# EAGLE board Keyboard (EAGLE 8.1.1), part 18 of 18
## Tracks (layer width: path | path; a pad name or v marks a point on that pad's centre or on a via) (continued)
S$18700 (continued)
  Bottom 0.381: 271.04,2.46 269.52,3.98
S$18701
  Bottom 0.381: 294.75,2.46 288.9,2.46
S$18702
  Bottom 0.381: 288.9,2.46 287.38,3.98
S$18703
  Bottom 0.381: 315.08,12.62 315.08,13.89
S$18704
  Bottom 0.381: 315.08,13.89 313.34,15.63
S$18705
  Bottom 0.381: 313.34,15.63 313.34,15.89
S$18706
  Bottom 0.381: 315.08,88.82 315.08,87.55
S$18707
  Bottom 0.381: 315.08,87.55 312.29,84.76
S$18708
  Bottom 0.381: 312.29,84.76 312.29,76.47
S$18709
  Bottom 0.381: 312.29,76.47 313.34,75.42
S$18710
  Bottom 0.381: 296.03,69.77 296.03,71.04
S$18711
  Bottom 0.381: 296.03,71.04 294.29,72.77
S$18712
  Bottom 0.381: 294.29,72.77 294.29,73.04
S$18713
  Bottom 0.381: 296.03,12.62 296.03,13.89
S$18714
  Bottom 0.381: 296.03,13.89 294.29,15.63
S$18715
  Bottom 0.381: 294.29,15.63 294.29,15.89
S$18716
  Bottom 0.381: 315.08,69.77 315.08,71.04
S$18717
  Bottom 0.381: 315.08,71.04 313.34,72.77
S$18718
  Bottom 0.381: 313.34,72.77 313.34,73.04
S$18719
  Bottom 0.381: 193.31,23.03 198.78,23.03
S$18720
  Bottom 0.381: 198.78,23.03 200.28,21.53
S$18721
  Bottom 0.381: 294.76,21.51 290.09,21.51
S$18722
  Bottom 0.381: 290.09,21.51 288.56,23.03
S$18723
  Bottom 0.381: 268.22,69.78 269.49,69.78
S$18724
  Bottom 0.381: 269.49,69.78 269.49,69.22
S$18725
  Bottom 0.381: 269.49,69.22 270.2,68.51
S$18726
  Bottom 0.381: 270.2,68.51 277.86,68.51
S$18727
  Bottom 0.381: 179.02,61.13 184.49,61.13
S$18728
  Bottom 0.381: 184.49,61.13 185.99,59.63
S$18729
  Bottom 0.381: 254.04,58.75 244.01,58.75
S$18730
  Bottom 0.381: 244.01,58.75 243.14,59.62
S$18731
  Bottom 0.381: 174.26,30.65 168.98,30.65
S$18732
  Bottom 0.381: 168.98,30.65 166.68,32.95
S$18733
  Bottom 0.381: 166.68,32.95 165.41,32.95
S$18734
  Bottom 0.381: 165.41,32.95 164.71,32.24
S$18735
  Bottom 0.381: 164.71,32.24 164.71,30.54
S$18736
  Bottom 0.381: 164.71,30.54 164.45,30.28
S$18737
  Bottom 0.381: 164.45,30.28 155.57,30.28
S$18738
  Bottom 0.381: 155.57,30.28 155.21,30.65
S$18739
  Bottom 0.381: 98.05,30.65 97.7,30.29
S$18740
  Bottom 0.381: 97.7,30.29 79.35,30.29
S$18741
  Bottom 0.381: 79.35,30.29 79,30.65
S$18742
  Bottom 0.381: 136.15,30.65 135.77,30.26
S$18743
  Bottom 0.381: 135.77,30.26 117.49,30.26
S$18744
  Bottom 0.381: 117.49,30.26 117.1,30.65
S$18745
  Bottom 0.381: 155.21,23.03 160.68,23.03
S$18746
  Bottom 0.381: 160.68,23.03 162.18,21.52
S$18747
  Bottom 0.381: 144.4,31.69 144.4,32.96
S$18748
  Bottom 0.381: 144.4,32.96 143.85,32.96
S$18749
  Bottom 0.381: 143.85,32.96 141.87,34.94
S$18750
  Bottom 0.381: 294.75,59.61 290.09,59.61
S$18751
  Bottom 0.381: 290.09,59.61 288.57,61.13
S$18752
  Bottom 0.381: 294.75,78.66 293,78.66
S$18753
  Bottom 0.381: 293,78.66 287.39,73.04
S$18754
  Bottom 0.381: 283.78,80.82 286.22,83.26
S$18755
  Bottom 0.381: 286.22,83.26 286.22,83.42
S$18756
  Bottom 0.381: 45.66,61.13 51.14,61.13
S$18757
  Bottom 0.381: 51.14,61.13 52.64,59.63
S$18758
  Bottom 0.381: 69.47,42.08 74.95,42.08
S$18759
  Bottom 0.381: 74.95,42.08 76.45,40.57
S$18760
  Bottom 0.381: 313.8,2.46 298.98,2.46
S$18761
  Bottom 0.381: 298.98,2.46 298.55,2.89
S$18762
  Bottom 0.381: 298.55,2.89 297.76,2.89
S$18763
  Bottom 0.381: 297.76,2.89 296.91,3.74
S$18764
  Bottom 0.381: 296.91,3.74 296.91,3.98
S$18765
  Bottom 0.381: 296.91,3.98 289.76,3.98
S$18766
  Bottom 0.381: 297.57,77.69 297,77.12
S$18767
  Bottom 0.381: 297,77.12 293.85,77.12
S$18768
  Bottom 0.381: 293.85,77.12 289.77,73.04
S$18769
  Bottom 0.381: 307.63,61.13 309.14,59.61
S$18770
  Bottom 0.381: 309.14,59.61 309.35,59.61
S$18771
  Bottom 0.381: 50.42,42.08 55.9,42.08
S$18772
  Bottom 0.381: 55.9,42.08 57.41,40.57
S$18773
  Bottom 0.381: 25.42,2.78 23.62,0.99
S$18774
  Bottom 0.381: 23.62,0.99 8.88,0.99
S$18775
  Bottom 0.381: 8.88,0.99 7.4,2.47
S$18776
  Bottom 0.381: 246.8,12.63 248.07,12.63
S$18777
  Bottom 0.381: 248.07,12.63 248.07,12
S$18778
  Bottom 0.381: 248.07,12 248.7,11.36
S$18779
  Bottom 0.381: 248.7,11.36 255.24,11.36
S$18780
  Bottom 0.381: 255.24,11.36 256.43,12.55
S$18781
  Bottom 0.381: 280.76,26.2 281.42,25.55
S$18782
  Bottom 0.381: 281.42,25.55 281.42,22.81
S$18783
  Bottom 0.381: 272.86,24.62 272.09,25.39
S$18784
  Bottom 0.381: 272.09,25.39 272.09,29.48
S$18785
  Bottom 0.381: 272.09,29.48 272.2,29.6
S$18786
  Bottom 0.381: 272.2,29.6 277.37,29.6
S$18787
  Bottom 0.381: 277.37,29.6 280.76,26.2
S$18788
  Bottom 0.381: 280.76,26.2 284.99,30.43
S$18789
  Bottom 0.381: 272.86,23.03 272.86,24.62
S$18790
  Bottom 0.381: 220.6,31.69 220.6,32.96
S$18791
  Bottom 0.381: 220.6,32.96 220.06,32.96
S$18792
  Bottom 0.381: 220.06,32.96 218.08,34.94
S$18793
  Bottom 0.381: 201.55,31.69 201.55,32.96
S$18794
  Bottom 0.381: 201.55,32.96 201.01,32.96
S$18795
  Bottom 0.381: 201.01,32.96 199.03,34.94
S$18796
  Bottom 0.381: 225.36,69.78 225.36,71.05
S$18797
  Bottom 0.381: 225.36,71.05 224.83,71.05
S$18798
  Bottom 0.381: 224.83,71.05 222.84,73.04
S$18799
  Bottom 0.381: 39.62,50.74 39.62,52.01
S$18800
  Bottom 0.381: 39.62,52.01 39.07,52.01
S$18801
  Bottom 0.381: 39.07,52.01 37.09,53.99
S$18802
  Bottom 0.381: 82.49,88.83 82.49,87.56
S$18803
  Bottom 0.381: 82.49,87.56 79.64,84.71
S$18804
  Bottom 0.381: 79.64,84.71 79.64,75.73
S$18805
  Bottom 0.381: 79.64,75.73 79.95,75.42
S$18806
  Bottom 0.381: 87.25,31.68 87.25,32.95
S$18807
  Bottom 0.381: 84.72,34.94 86.7,32.95
S$18808
  Bottom 0.381: 86.7,32.95 87.25,32.95
S$18809
  Bottom 0.381: 77.72,50.73 77.72,52
S$18810
  Bottom 0.381: 77.72,52 77.18,52
S$18811
  Bottom 0.381: 77.18,52 75.19,53.99
S$18812
  Bottom 0.381: 164.74,42.08 170.2,42.08
S$18813
  Bottom 0.381: 170.2,42.08 171.7,40.57
S$18814
  Bottom 0.381: 183.79,42.08 189.25,42.08
S$18815
  Bottom 0.381: 189.25,42.08 190.75,40.58
S$18816
  Bottom 0.381: 211.07,50.74 211.07,52.01
S$18817
  Bottom 0.381: 211.07,52.01 210.54,52.01
S$18818
  Bottom 0.381: 210.54,52.01 208.55,53.98
S$18819
  Bottom 0.381: 221.89,42.08 223.39,40.58
S$18820
  Bottom 0.381: 223.39,40.58 228.85,40.58
S$18821
  Bottom 0.381: 261.08,50.73 261.08,52
S$18822
  Bottom 0.381: 261.08,52 260.56,52
S$18823
  Bottom 0.381: 260.56,52 258.57,53.99
S$18824
  Bottom 0.381: 49.15,31.69 49.15,32.96
S$18825
  Bottom 0.381: 49.15,32.96 48.59,32.96
S$18826
  Bottom 0.381: 48.59,32.96 46.61,34.94
S$18827
  Bottom 0.381: 42.09,23.03 46.38,23.03
S$18828
  Bottom 0.381: 46.38,23.03 47.88,21.53
S$18829
  Bottom 0.381: 68.2,31.68 68.2,32.95
S$18830
  Bottom 0.381: 68.2,32.95 67.65,32.95
S$18831
  Bottom 0.381: 67.65,32.95 65.66,34.94
S$18832
  Bottom 0.381: 59.94,23.03 65.42,23.03
S$18833
  Bottom 0.381: 65.42,23.03 66.93,21.52
S$18834
  Bottom 0.381: 153.92,50.73 153.92,52
S$18835
  Bottom 0.381: 153.92,52 153.39,52
S$18836
  Bottom 0.381: 153.39,52 151.4,53.99
S$18837
  Bottom 0.381: 126.62,42.08 132.1,42.08
S$18838
  Bottom 0.381: 132.1,42.08 133.6,40.57
S$18839
  Bottom 0.381: 79,23.03 84.47,23.03
S$18840
  Bottom 0.381: 84.47,23.03 85.98,21.52
S$18841
  Bottom 0.381: 44.47,3.98 43.34,5.11
S$18842
  Bottom 0.381: 43.34,5.11 41.17,5.11
S$18843
  Bottom 0.381: 41.17,5.11 38.54,2.48
S$18844
  Bottom 0.381: 38.54,2.48 31.21,2.48
S$18845
  Bottom 0.381: 56.29,12.64 56.29,13.91
S$18846
  Bottom 0.381: 56.29,13.91 55.74,13.91
S$18847
  Bottom 0.381: 55.74,13.91 53.76,15.89
S$18848
  Bottom 0.381: 49.23,3.98 53.52,3.98
S$18849
  Bottom 0.381: 53.52,3.98 55.02,2.48
S$18850
  Bottom 0.381: 127.73,12.63 127.73,13.9
S$18851
  Bottom 0.381: 127.73,13.9 127.19,13.9
S$18852
  Bottom 0.381: 127.19,13.9 125.2,15.88
S$18853
  Bottom 0.381: 121.87,15.88 121.87,7.07
S$18854
  Bottom 0.381: 121.87,7.07 126.46,2.47
S$18855
  Bottom 0.381: 199.17,12.63 199.17,13.9
S$18856
  Bottom 0.381: 199.17,13.9 198.63,13.9
S$18857
  Bottom 0.381: 198.63,13.9 196.65,15.88
S$18858
  Bottom 0.381: 193.31,15.88 193.31,7.06
S$18859
  Bottom 0.381: 193.31,7.06 197.9,2.47
S$18860
  Bottom 0.381: 222.98,12.63 222.98,13.9
S$18861
  Bottom 0.381: 222.98,13.9 222.45,13.9
S$18862
  Bottom 0.381: 222.45,13.9 220.46,15.88
S$18863
  Bottom 0.381: 238.56,3.98 244.03,3.98
S$18864
  Bottom 0.381: 244.03,3.98 245.53,2.47
S$18865
  Bottom 0.381: 6.29,88.83 6.29,87.56
S$18866
  Bottom 0.381: 6.29,87.56 3.44,84.71
S$18867
  Bottom 0.381: 3.44,84.71 3.44,75.72
S$18868
  Bottom 0.381: 3.44,75.72 3.75,75.42
S$18869
  Bottom 0.381: 22.8,75.42 22.36,75.85
S$18870
  Bottom 0.381: 22.36,75.85 22.36,76.22
S$18871
  Bottom 0.381: 22.36,76.22 21.8,76.78
S$18872
  Bottom 0.381: 21.8,76.78 21.8,80.72
S$18873
  Bottom 0.381: 21.8,80.72 22.13,81.05
S$18874
  Bottom 0.381: 22.13,81.05 22.36,81.05
S$18875
  Bottom 0.381: 22.36,81.05 22.36,84.59
S$18876
  Bottom 0.381: 22.36,84.59 25.34,87.56
S$18877
  Bottom 0.381: 25.34,88.83 25.34,87.56
S$18878
  Bottom 0.381: 44.39,88.84 44.39,87.57
S$18879
  Bottom 0.381: 44.39,87.57 41.54,84.72
S$18880
  Bottom 0.381: 41.54,84.72 41.54,75.72
S$18881
  Bottom 0.381: 41.54,75.72 41.85,75.42
S$18882
  Bottom 0.381: 63.44,88.84 63.44,87.57
S$18883
  Bottom 0.381: 63.44,87.57 60.59,84.72
S$18884
  Bottom 0.381: 60.59,84.72 60.59,75.73
S$18885
  Bottom 0.381: 60.59,75.73 60.9,75.42
S$18886
  Bottom 0.381: 101.54,88.84 101.54,87.57
S$18887
  Bottom 0.381: 101.54,87.57 98.51,84.54
S$18888
  Bottom 0.381: 98.51,84.54 98.51,75.91
S$18889
  Bottom 0.381: 98.51,75.91 99.01,75.42
S$18890
  Bottom 0.381: 120.59,88.84 120.59,87.57
S$18891
  Bottom 0.381: 120.59,87.57 117.74,84.72
S$18892
  Bottom 0.381: 117.74,84.72 117.74,75.73
S$18893
  Bottom 0.381: 117.74,75.73 118.06,75.42
S$18894
  Bottom 0.381: 139.64,88.84 139.64,87.57
S$18895
  Bottom 0.381: 139.64,87.57 136.68,84.61
S$18896
  Bottom 0.381: 136.68,84.61 136.68,75.84
S$18897
  Bottom 0.381: 136.68,75.84 137.11,75.42
S$18898
  Bottom 0.381: 158.69,88.84 158.69,87.57
S$18899
  Bottom 0.381: 158.69,87.57 155.78,84.66
S$18900
  Bottom 0.381: 155.78,84.66 155.78,75.8
S$18901
  Bottom 0.381: 155.78,75.8 156.16,75.42
S$18902
  Bottom 0.381: 177.74,88.84 177.74,87.57
S$18903
  Bottom 0.381: 177.74,87.57 174.93,84.76
S$18904
  Bottom 0.381: 174.93,84.76 174.93,75.7
S$18905
  Bottom 0.381: 174.93,75.7 175.22,75.42
S$18906
  Bottom 0.381: 196.79,88.83 196.79,87.56
S$18907
  Bottom 0.381: 196.79,87.56 193.87,84.65
S$18908
  Bottom 0.381: 193.87,84.65 193.87,75.81
S$18909
  Bottom 0.381: 193.87,75.81 194.27,75.42
S$18910
  Bottom 0.381: 215.84,88.83 215.84,87.56
S$18911
  Bottom 0.381: 215.84,87.56 213,84.73
S$18912
  Bottom 0.381: 213,84.73 213,75.73
S$18913
  Bottom 0.381: 213,75.73 213.32,75.42
S$18914
  Bottom 0.381: 234.89,88.83 234.89,87.56
S$18915
  Bottom 0.381: 234.89,87.56 232.05,84.73
S$18916
  Bottom 0.381: 232.05,84.73 232.05,75.73
S$18917
  Bottom 0.381: 232.05,75.73 232.37,75.42
S$18918
  Bottom 0.381: 266.73,87.37 267.19,86.9
S$18919
  Bottom 0.381: 267.19,86.9 267.19,82.69
S$18920
  Bottom 0.381: 267.19,82.69 264.69,80.19
S$18921
  Bottom 0.381: 264.69,80.19 264.69,73.93
S$18922
  Bottom 0.381: 264.69,73.93 261.43,70.66
S$18923
  Bottom 0.381: 257.61,68.27 257.61,74.09
S$18924
  Bottom 0.381: 257.61,74.09 262.19,78.67
S$18925
  Bottom 0.381: 11.05,69.79 11.05,71.06
S$18926
  Bottom 0.381: 11.05,71.06 10.49,71.06
S$18927
  Bottom 0.381: 10.49,71.06 8.51,73.04
S$18928
  Bottom 0.381: 34.86,69.79 34.86,71.06
S$18929
  Bottom 0.381: 34.86,71.06 34.31,71.06
S$18930
  Bottom 0.381: 34.31,71.06 32.32,73.04
S$18931
  Bottom 0.381: 26.61,61.13 32.09,61.13
S$18932
  Bottom 0.381: 32.09,61.13 33.59,59.63
S$18933
  Bottom 0.381: 53.91,69.79 53.91,71.06
S$18934
  Bottom 0.381: 53.91,71.06 53.37,71.06
S$18935
  Bottom 0.381: 53.37,71.06 51.38,73.05
S$18936
  Bottom 0.381: 92.01,69.78 92.01,71.05
S$18937
  Bottom 0.381: 92.01,71.05 91.47,71.05
S$18938
  Bottom 0.381: 91.47,71.05 89.48,73.04
S$18939
  Bottom 0.381: 111.06,69.78 111.06,71.05
S$18940
  Bottom 0.381: 111.06,71.05 110.52,71.05
S$18941
  Bottom 0.381: 110.52,71.05 108.53,73.04
S$18942
  Bottom 0.381: 130.11,69.78 130.11,71.05
S$18943
  Bottom 0.381: 130.11,71.05 129.57,71.05
S$18944
  Bottom 0.381: 129.57,71.05 127.58,73.04
S$18945
  Bottom 0.381: 149.16,69.78 149.16,71.05
S$18946
  Bottom 0.381: 149.16,71.05 148.62,71.05
S$18947
  Bottom 0.381: 148.62,71.05 146.63,73.04
S$18948
  Bottom 0.381: 244.41,69.78 244.41,71.05
S$18949
  Bottom 0.381: 244.41,71.05 243.88,71.05
S$18950
  Bottom 0.381: 243.88,71.05 241.89,73.04
S$18951
  Bottom 0.381: 58.68,50.73 58.68,52
S$18952
  Bottom 0.381: 58.68,52 58.12,52
S$18953
  Bottom 0.381: 58.12,52 56.14,53.98
S$18954
  Bottom 0.381: 258.8,13.5 258.8,17.77
S$18955
  Bottom 0.381: 258.8,17.77 255.05,21.52
S$18956
  Bottom 0.381: 224.09,59.62 222.59,61.13
S$18957
  Bottom 0.381: 222.59,61.13 217.12,61.13
S$18958
  Bottom 0.381: 125.35,31.68 125.35,32.95
S$18959
  Bottom 0.381: 125.35,32.95 124.81,32.95
S$18960
  Bottom 0.381: 124.81,32.95 122.82,34.94
S$18961
  Bottom 0.381: 163.45,31.68 163.45,32.95
S$18962
  Bottom 0.381: 163.45,32.95 162.91,32.95
S$18963
  Bottom 0.381: 162.91,32.95 160.93,34.94
S$18964
  Bottom 0.381: 230.23,22.79 233.03,22.79
S$18965
  Bottom 0.381: 233.03,22.79 241.93,31.68
S$18966
  Bottom 0.381: 189.74,80.18 188.23,78.68
S$18967
  Bottom 0.381: 188.23,78.68 176.47,78.68
S$18968
  Bottom 0.381: 64.71,61.13 70.19,61.13
S$18969
  Bottom 0.381: 70.19,61.13 71.69,59.62
S$18970
  Bottom 0.381: 206.31,69.78 206.31,71.05
S$18971
  Bottom 0.381: 206.31,71.05 205.78,71.05
S$18972
  Bottom 0.381: 205.78,71.05 203.79,73.04
S$18973
  Bottom 0.381: 72.96,69.78 72.96,71.05
S$18974
  Bottom 0.381: 72.96,71.05 72.42,71.05
S$18975
  Bottom 0.381: 72.42,71.05 70.43,73.04
S$18976
  Bottom 0.381: 134.87,50.73 134.87,52
S$18977
  Bottom 0.381: 134.87,52 134.34,52
S$18978
  Bottom 0.381: 134.34,52 132.35,53.99
S$18979
  Bottom 0.381: 172.97,50.73 172.97,52
S$18980
  Bottom 0.381: 172.97,52 172.44,52
S$18981
  Bottom 0.381: 172.44,52 170.45,53.98
S$18982
  Bottom 0.381: 96.77,50.73 96.77,52
S$18983
  Bottom 0.381: 96.77,52 96.22,52
S$18984
  Bottom 0.381: 96.22,52 94.24,53.98
S$18985
  Bottom 0.381: 106.3,31.68 106.3,32.95
S$18986
  Bottom 0.381: 106.3,32.95 105.76,32.95
S$18987
  Bottom 0.381: 105.76,32.95 103.77,34.94
S$18988
  Bottom 0.381: 98.05,23.03 103.53,23.03
S$18989
  Bottom 0.381: 103.53,23.03 105.03,21.52
S$18990
  Bottom 0.381: 8.67,12.63 7.4,12.63
S$18991
  Bottom 0.381: 7.4,12.63 7.4,11.91
S$18992
  Bottom 0.381: 7.4,11.91 1.6,6.12
S$18993
  Bottom 0.381: 37.33,80.18 36.17,81.33
S$18994
  Bottom 0.381: 36.17,81.33 34.14,81.33
S$18995
  Bottom 0.381: 34.14,81.33 31.48,78.67
S$18996
  Bottom 0.381: 31.48,78.67 24.07,78.67
S$18997
  Bottom 0.381: 168.21,69.78 168.21,71.05
S$18998
  Bottom 0.381: 168.21,71.05 167.68,71.05
S$18999
  Bottom 0.381: 167.68,71.05 165.69,73.04
S$19000
  Bottom 0.381: 187.26,69.79 187.26,71.06
S$19001
  Bottom 0.381: 187.26,71.06 186.73,71.06
S$19002
  Bottom 0.381: 186.73,71.06 184.74,73.04
S$19003
  Bottom 0.381: 198.07,61.13 203.53,61.13
S$19004
  Bottom 0.381: 203.53,61.13 205.04,59.62
S$19005
  Bottom 0.381: 226.65,80.18 226.65,82.51
S$19006
  Bottom 0.381: 226.65,82.51 218.94,90.22
S$19007
  Bottom 0.381: 218.94,90.22 217.98,90.22
S$19008
  Bottom 0.381: 217.98,90.22 217.09,89.33
S$19009
  Bottom 0.381: 217.09,89.33 217.09,87.78
S$19010
  Bottom 0.381: 217.09,87.78 214.57,85.26
S$19011
  Bottom 0.381: 214.57,85.26 214.57,78.67
S$19012
  Bottom 0.635: 27.8,46.51 33.76,40.55
S$19013
  Bottom 0.635: 33.76,40.55 34.03,40.55
S$19014
  Bottom 0.635: 34.03,40.55 45.45,29.13
S$19015
  Bottom 0.203: 321.58,54.3 322.88,53.92
S$19016
  Bottom 0.203: 321.58,53.55 322.88,53.92
S$19017
  Bottom 0.203: 321.58,53.55 322.88,53.19
S$19018
  Bottom 0.203: 321.58,52.82 322.88,53.19
S$19019
  Bottom 0.203: 321.58,52.2 322.88,51.83
S$19020
  Bottom 0.203: 321.58,51.47 322.88,51.83
S$19021
  Bottom 0.203: 321.58,51.47 322.88,51.09
S$19022
  Bottom 0.203: 321.58,50.73 322.88,51.09
S$19023
  Bottom 0.203: 321.58,50.12 322.88,49.75
S$19024
  Bottom 0.203: 321.58,49.38 322.88,49.75
S$19025
  Bottom 0.203: 321.58,49.38 322.88,49.01
S$19026
  Bottom 0.203: 321.58,48.64 322.88,49.01
S$19027
  Bottom 0.203: 322.41,47.94 322.51,48.03
S$19028
  Bottom 0.203: 322.51,48.03 322.6,47.94
S$19029
  Bottom 0.203: 322.6,47.94 322.51,47.84
S$19030
  Bottom 0.203: 322.51,47.84 322.41,47.94
S$19031
  Bottom 0.203: 321.21,46.13 321.03,46.22
S$19032
  Bottom 0.203: 321.03,46.22 320.94,46.5
S$19033
  Bottom 0.203: 320.94,46.5 320.94,46.68
S$19034
  Bottom 0.203: 320.94,46.68 321.03,46.96
S$19035
  Bottom 0.203: 321.03,46.96 321.31,47.14
S$19036
  Bottom 0.203: 321.31,47.14 321.77,47.23
S$19037
  Bottom 0.203: 321.77,47.23 322.23,47.23
S$19038
  Bottom 0.203: 322.23,47.23 322.6,47.14
S$19039
  Bottom 0.203: 322.6,47.14 322.78,46.96
S$19040
  Bottom 0.203: 322.78,46.96 322.88,46.68
S$19041
  Bottom 0.203: 322.88,46.68 322.88,46.59
S$19042
  Bottom 0.203: 322.88,46.59 322.78,46.31
S$19043
  Bottom 0.203: 322.78,46.31 322.6,46.13
S$19044
  Bottom 0.203: 322.6,46.13 322.32,46.04
S$19045
  Bottom 0.203: 322.32,46.04 322.23,46.04
S$19046
  Bottom 0.203: 322.23,46.04 321.95,46.13
S$19047
  Bottom 0.203: 321.95,46.13 321.77,46.31
S$19048
  Bottom 0.203: 321.77,46.31 321.68,46.59
S$19049
  Bottom 0.203: 321.68,46.59 321.68,46.68
S$19050
  Bottom 0.203: 321.68,46.68 321.77,46.96
S$19051
  Bottom 0.203: 321.77,46.96 321.95,47.14
S$19052
  Bottom 0.203: 321.95,47.14 322.23,47.23
S$19053
  Bottom 0.203: 320.94,44.87 321.03,45.15
S$19054
  Bottom 0.203: 321.03,45.15 321.31,45.33
S$19055
  Bottom 0.203: 321.31,45.33 321.77,45.42
S$19056
  Bottom 0.203: 321.77,45.42 322.04,45.42
S$19057
  Bottom 0.203: 322.04,45.42 322.51,45.33
S$19058
  Bottom 0.203: 322.51,45.33 322.78,45.15
S$19059
  Bottom 0.203: 322.78,45.15 322.88,44.87
S$19060
  Bottom 0.203: 322.88,44.87 322.88,44.69
S$19061
  Bottom 0.203: 322.88,44.69 322.78,44.41
S$19062
  Bottom 0.203: 322.78,44.41 322.51,44.22
S$19063
  Bottom 0.203: 322.51,44.22 322.04,44.13
S$19064
  Bottom 0.203: 322.04,44.13 321.77,44.13
S$19065
  Bottom 0.203: 321.77,44.13 321.31,44.22
S$19066
  Bottom 0.203: 321.31,44.22 321.03,44.41
S$19067
  Bottom 0.203: 321.03,44.41 320.94,44.69
S$19068
  Bottom 0.203: 320.94,44.69 320.94,44.87
S$19069
  Bottom 0.203: 321.58,43.52 323.52,43.52
S$19070
  Bottom 0.203: 321.86,43.52 321.68,43.34
S$19071
  Bottom 0.203: 321.68,43.34 321.58,43.15
S$19072
  Bottom 0.203: 321.58,43.15 321.58,42.87
S$19073
  Bottom 0.203: 321.58,42.87 321.68,42.69
S$19074
  Bottom 0.203: 321.68,42.69 321.86,42.51
S$19075
  Bottom 0.203: 321.86,42.51 322.14,42.41
S$19076
  Bottom 0.203: 322.14,42.41 322.32,42.41
S$19077
  Bottom 0.203: 322.32,42.41 322.6,42.51
S$19078
  Bottom 0.203: 322.6,42.51 322.78,42.69
S$19079
  Bottom 0.203: 322.78,42.69 322.88,42.87
S$19080
  Bottom 0.203: 322.88,42.87 322.88,43.15
S$19081
  Bottom 0.203: 322.88,43.15 322.78,43.34
S$19082
  Bottom 0.203: 322.78,43.34 322.6,43.52
S$19083
  Bottom 0.203: 322.14,41.8 322.14,40.7
S$19084
  Bottom 0.203: 322.14,40.7 321.95,40.7
S$19085
  Bottom 0.203: 321.95,40.7 321.77,40.78
S$19086
  Bottom 0.203: 321.77,40.78 321.68,40.88
S$19087
  Bottom 0.203: 321.68,40.88 321.58,41.06
S$19088
  Bottom 0.203: 321.58,41.06 321.58,41.34
S$19089
  Bottom 0.203: 321.58,41.34 321.68,41.53
S$19090
  Bottom 0.203: 321.68,41.53 321.86,41.71
S$19091
  Bottom 0.203: 321.86,41.71 322.14,41.8
S$19092
  Bottom 0.203: 322.14,41.8 322.32,41.8
S$19093
  Bottom 0.203: 322.32,41.8 322.6,41.71
S$19094
  Bottom 0.203: 322.6,41.71 322.78,41.53
S$19095
  Bottom 0.203: 322.78,41.53 322.88,41.34
S$19096
  Bottom 0.203: 322.88,41.34 322.88,41.06
S$19097
  Bottom 0.203: 322.88,41.06 322.78,40.88
S$19098
  Bottom 0.203: 322.78,40.88 322.6,40.7
S$19099
  Bottom 0.203: 321.58,40.09 322.88,40.09
S$19100
  Bottom 0.203: 322.14,40.09 321.86,39.99
S$19101
  Bottom 0.203: 321.86,39.99 321.68,39.81
S$19102
  Bottom 0.203: 321.68,39.81 321.58,39.62
S$19103
  Bottom 0.203: 321.58,39.62 321.58,39.35
S$19104
  Bottom 0.203: 321.86,37.63 321.68,37.82
S$19105
  Bottom 0.203: 321.68,37.82 321.58,38
S$19106
  Bottom 0.203: 321.58,38 321.58,38.27
S$19107
  Bottom 0.203: 321.58,38.27 321.68,38.46
S$19108
  Bottom 0.203: 321.68,38.46 321.86,38.65
S$19109
  Bottom 0.203: 321.86,38.65 322.14,38.74
S$19110
  Bottom 0.203: 322.14,38.74 322.32,38.74
S$19111
  Bottom 0.203: 322.32,38.74 322.6,38.65
S$19112
  Bottom 0.203: 322.6,38.65 322.78,38.46
S$19113
  Bottom 0.203: 322.78,38.46 322.88,38.27
S$19114
  Bottom 0.203: 322.88,38.27 322.88,38
S$19115
  Bottom 0.203: 322.88,38 322.78,37.82
S$19116
  Bottom 0.203: 322.78,37.82 322.6,37.63
S$19117
  Bottom 0.203: 322.14,37.02 322.14,35.91
S$19118
  Bottom 0.203: 322.14,35.91 321.95,35.91
S$19119
  Bottom 0.203: 321.95,35.91 321.77,36.01
S$19120
  Bottom 0.203: 321.77,36.01 321.68,36.1
S$19121
  Bottom 0.203: 321.68,36.1 321.58,36.28
S$19122
  Bottom 0.203: 321.58,36.28 321.58,36.56
S$19123
  Bottom 0.203: 321.58,36.56 321.68,36.74
S$19124
  Bottom 0.203: 321.68,36.74 321.86,36.93
S$19125
  Bottom 0.203: 321.86,36.93 322.14,37.02
S$19126
  Bottom 0.203: 322.14,37.02 322.32,37.02
S$19127
  Bottom 0.203: 322.32,37.02 322.6,36.93
S$19128
  Bottom 0.203: 322.6,36.93 322.78,36.74
S$19129
  Bottom 0.203: 322.78,36.74 322.88,36.56
S$19130
  Bottom 0.203: 322.88,36.56 322.88,36.28
S$19131
  Bottom 0.203: 322.88,36.28 322.78,36.1
S$19132
  Bottom 0.203: 322.78,36.1 322.6,35.91
S$19133
  Bottom 0.203: 321.58,35.3 322.88,35.3
S$19134
  Bottom 0.203: 321.95,35.3 321.68,35.02
S$19135
  Bottom 0.203: 321.68,35.02 321.58,34.84
S$19136
  Bottom 0.203: 321.58,34.84 321.58,34.56
S$19137
  Bottom 0.203: 321.58,34.56 321.68,34.38
S$19138
  Bottom 0.203: 321.68,34.38 321.95,34.28
S$19139
  Bottom 0.203: 321.95,34.28 322.88,34.28
S$19140
  Bottom 0.203: 320.94,33.4 322.51,33.4
S$19141
  Bottom 0.203: 322.51,33.4 322.78,33.31
S$19142
  Bottom 0.203: 322.78,33.31 322.88,33.12
S$19143
  Bottom 0.203: 322.88,33.12 322.88,32.94
S$19144
  Bottom 0.203: 321.58,33.67 321.58,33.03
S$19145
  Bottom 0.203: 322.41,32.23 322.51,32.33
S$19146
  Bottom 0.203: 322.51,32.33 322.6,32.23
S$19147
  Bottom 0.203: 322.6,32.23 322.51,32.14
S$19148
  Bottom 0.203: 322.51,32.14 322.41,32.23
S$19149
  Bottom 0.203: 321.86,30.42 321.68,30.61
S$19150
  Bottom 0.203: 321.68,30.61 321.58,30.8
S$19151
  Bottom 0.203: 321.58,30.8 321.58,31.07
S$19152
  Bottom 0.203: 321.58,31.07 321.68,31.26
S$19153
  Bottom 0.203: 321.68,31.26 321.86,31.44
S$19154
  Bottom 0.203: 321.86,31.44 322.14,31.53
S$19155
  Bottom 0.203: 322.14,31.53 322.32,31.53
S$19156
  Bottom 0.203: 322.32,31.53 322.6,31.44
S$19157
  Bottom 0.203: 322.6,31.44 322.78,31.26
S$19158
  Bottom 0.203: 322.78,31.26 322.88,31.07
S$19159
  Bottom 0.203: 322.88,31.07 322.88,30.8
S$19160
  Bottom 0.203: 322.88,30.8 322.78,30.61
S$19161
  Bottom 0.203: 322.78,30.61 322.6,30.42
S$19162
  Bottom 0.203: 320.94,29.82 322.88,29.82
S$19163
  Bottom 0.203: 321.58,29.2 322.51,29.2
S$19164
  Bottom 0.203: 322.51,29.2 322.78,29.12
S$19165
  Bottom 0.203: 322.78,29.12 322.88,28.93
S$19166
  Bottom 0.203: 322.88,28.93 322.88,28.65
S$19167
  Bottom 0.203: 322.88,28.65 322.78,28.47
S$19168
  Bottom 0.203: 322.78,28.47 322.51,28.19
S$19169
  Bottom 0.203: 321.58,28.19 322.88,28.19
S$19170
  Bottom 0.203: 320.94,27.58 322.88,27.58
S$19171
  Bottom 0.203: 321.86,27.58 321.68,27.4
S$19172
  Bottom 0.203: 321.68,27.4 321.58,27.21
S$19173
  Bottom 0.203: 321.58,27.21 321.58,26.93
S$19174
  Bottom 0.203: 321.58,26.93 321.68,26.75
S$19175
  Bottom 0.203: 321.68,26.75 321.86,26.56
S$19176
  Bottom 0.203: 321.86,26.56 322.14,26.47
S$19177
  Bottom 0.203: 322.14,26.47 322.32,26.47
S$19178
  Bottom 0.203: 322.32,26.47 322.6,26.56
S$19179
  Bottom 0.203: 322.6,26.56 322.78,26.75
S$19180
  Bottom 0.203: 322.78,26.75 322.88,26.93
S$19181
  Bottom 0.203: 322.88,26.93 322.88,27.21
S$19182
  Bottom 0.203: 322.88,27.21 322.78,27.4
S$19183
  Bottom 0.203: 322.78,27.4 322.6,27.58
(copper drawn outside any net)
  shapes: Bottom area x172, Bottom circle x1242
